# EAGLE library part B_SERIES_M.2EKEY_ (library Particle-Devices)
Particle B Series SoM 3042 M.2 Connector with E Key Width = 30mm Length = 42mm Height = 4.2mm Key = E
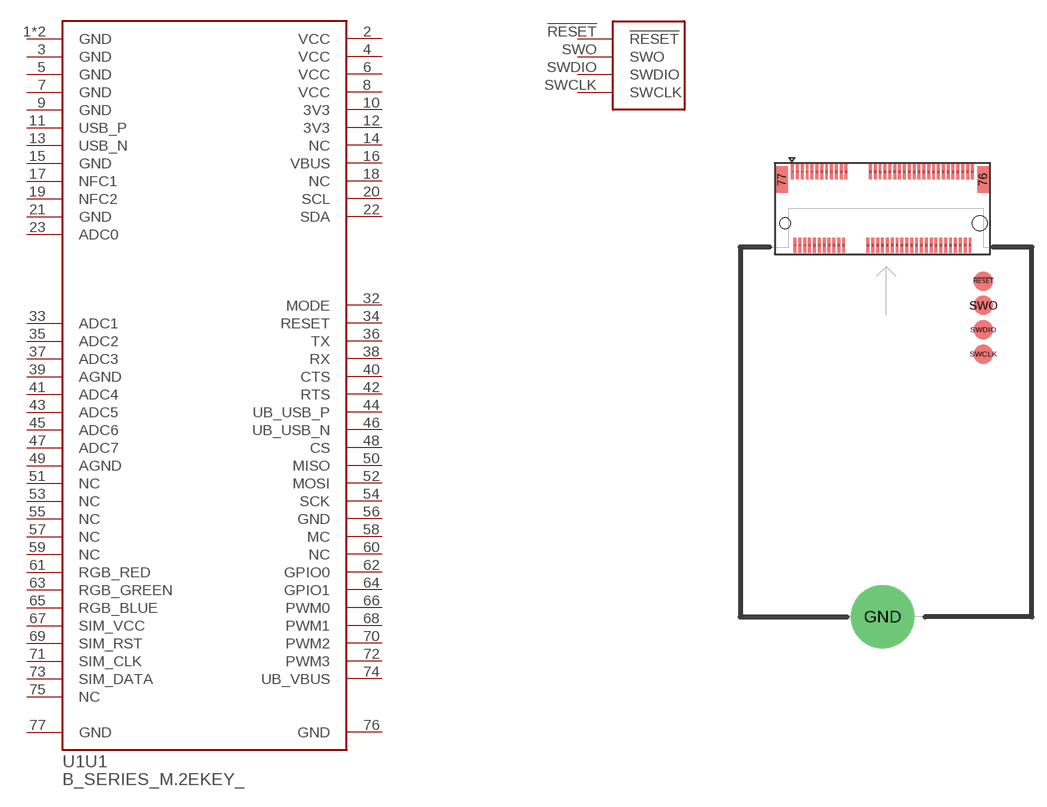
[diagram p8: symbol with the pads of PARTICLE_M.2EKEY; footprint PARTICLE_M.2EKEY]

Designator prefix U1; gates U1=B_SERIES_M.2EKEY G$1=B_SERIES_SWD

## B_SERIES_M.2EKEY_3042  [PARTICLE_M.2EKEY]
1  U1:GND  pwr
2  U1:VCC  pwr
3  U1:GND  pwr
4  U1:VCC  pwr
5  U1:GND  pwr
6  U1:VCC  pwr
7  U1:GND  pwr
8  U1:VCC  pwr
9  U1:GND  pwr
10  U1:3V3  pwr
11  U1:USB_P
12  U1:3V3  pwr
13  U1:USB_N
14  U1:NC
15  U1:GND  pwr
16  U1:VBUS  pwr
17  U1:NFC1
18  U1:NC
19  U1:NFC2
20  U1:SCL
21  U1:GND  pwr
22  U1:SDA
23  U1:ADC0
32  U1:MODE
33  U1:ADC1
34  U1:RESET
35  U1:ADC2
36  U1:TX
37  U1:ADC3
38  U1:RX
39  U1:AGND  pwr
40  U1:CTS
41  U1:ADC4
42  U1:RTS
43  U1:ADC5
44  U1:UB_USB_P
45  U1:ADC6
46  U1:UB_USB_N
47  U1:ADC7
48  U1:CS
49  U1:AGND  pwr
50  U1:MISO
51  U1:NC
52  U1:MOSI
53  U1:NC
54  U1:SCK
55  U1:NC
56  U1:GND  pwr
57  U1:NC
58  U1:MC
59  U1:NC
60  U1:NC
61  U1:RGB_RED
62  U1:GPIO0
63  U1:RGB_GREEN
64  U1:GPIO1
65  U1:RGB_BLUE
66  U1:PWM0
67  U1:SIM_VCC  pwr
68  U1:PWM1
69  U1:SIM_RST
70  U1:PWM2
71  U1:SIM_CLK
72  U1:PWM3
73  U1:SIM_DATA
74  U1:UB_VBUS  pwr
75  U1:NC
76  U1:GND  pwr
77  U1:GND  pwr
!RESET  G$1:!RESET  sup
GND  U1:GND  pwr
SWCLK  G$1:SWCLK  sup
SWDIO  G$1:SWDIO  sup
SWO  G$1:SWO  sup

## Footprint PARTICLE_M.2EKEY (pad centres in mm)
3042 M.2 Connector with E Key Width = 30mm Length = 42mm Height = 4.2mm Key = E
smd 0.3 x 1.55: 1 -9.62,3.735; 2 -9.37,-3.815; 3 -9.12,3.735; 4 -8.87,-3.815; 5 -8.62,3.735; 6 -8.37,-3.815; 7 -8.12,3.735; 8 -7.87,-3.815; 9 -7.62,3.735; 10 -7.37,-3.815; 11 -7.12,3.735; 12 -6.87,-3.815; 13 -6.62,3.735; 14 -6.37,-3.815; 15 -6.12,3.735; 16 -5.87,-3.815; 17 -5.62,3.735; 18 -5.37,-3.815; 19 -5.12,3.735; 20 -4.87,-3.815; 21 -4.62,3.735; 22 -4.37,-3.815; 23 -4.12,3.735; 32 -1.87,-3.815; 33 -1.62,3.735; 34 -1.37,-3.815; 35 -1.12,3.735; 36 -0.87,-3.815; 37 -0.62,3.735; 38 -0.37,-3.815; 39 -0.12,3.735; 40 0.13,-3.815; 41 0.38,3.735; 42 0.63,-3.815; 43 0.88,3.735; 44 1.13,-3.815; 45 1.38,3.735; 46 1.63,-3.815; 47 1.88,3.735; 48 2.13,-3.815; 49 2.38,3.735; 50 2.63,-3.815; 51 2.88,3.735; 52 3.13,-3.815; 53 3.38,3.735; 54 3.63,-3.815; 55 3.88,3.735; 56 4.13,-3.815; 57 4.38,3.735; 58 4.63,-3.815; 59 4.88,3.735; 60 5.13,-3.815; 61 5.38,3.735; 62 5.63,-3.815; 63 5.88,3.735; 64 6.13,-3.815; 65 6.38,3.735; 66 6.63,-3.815; 67 6.88,3.735; 68 7.13,-3.815; 69 7.38,3.735; 70 7.63,-3.815; 71 7.88,3.735; 72 8.13,-3.815; 73 8.38,3.735; 74 8.63,-3.815; 75 8.88,3.735
smd 1.2 x 2.75: 76 9.98,2.96; 77 -10.72,2.96
smd 2 x 2: !RESET 10,-7.5; SWCLK 10,-15; SWDIO 10,-12.5; SWO 10,-10
drill 2.6 pad 6.5: GND -0.351,-42
hole 1.1 at -10.37,-1.54
hole 1.55 at 9.63,-1.54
